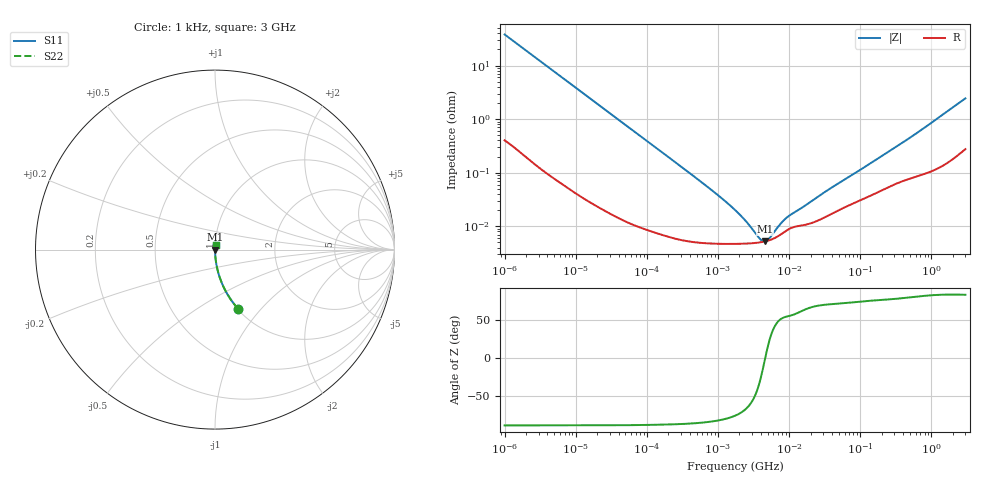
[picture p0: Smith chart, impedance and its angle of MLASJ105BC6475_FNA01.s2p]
! MLASJ105BC6475_FNA01  S-PARAMETER MODEL  ( Standard Model )
! Model Generated by TAIYO YUDEN Corporation (http://www.ty-top.com)
! Version 1.0
! TAIYO YUDEN Control No. 220601
! Copyright(c) 2013 TAIYO YUDEN CO.,LTD. All Rights Reserved.
! Product Description (link to TY-COMPAS)
! https://ds.yuden.co.jp/TYCOMPAS/or/detail?pn=MLASJ105BC6475MFNA01&u=M
! Products Name : Multilayer Ceramic Capacitors
! Characteristics :
!  Capacitance : 4.7 [uF] , Rated Voltage : 6.3 [V] , TCC : X6S
!  Case Size : 1.0 x 0.5 / 0.039 x 0.02 [mm/inch] , Thickness : 0.5 / 0.02 [mm/inch]
!  (Conditions: Temperature = 25 [degC] , DC Bias Voltage = 0 [V])
! External Node Assignments :
!  1  o---| |---o  2
! GND o---------o GND
! Frequency Range : 1kHz  -  3GHz  [ 401 STEP ]
# MHZ S RI R 50
! Freq[MHz].  S11 Real  S11 Imag  S21 Real  S21 Imag  S12 Real  S12 Imag  S22 Real  S22 Imag
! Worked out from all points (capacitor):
!   401 points, 1 kHz to 3 GHz, reference 50 ohm
!   read as one part in series: C = 4.18 uF near 1.077 kHz
!   lowest |Z| = 5.21 mohm at 4.566 MHz (marker M1)
!   series resonance near 4.61 MHz, so ESL is about 280 pH
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0.001  0.1285 -0.3294  0.8715 0.3294  0.8715 0.3294  0.1285 -0.3294
0.001685  0.0507 -0.2142  0.9493 0.2142  0.9493 0.2142  0.0507 -0.2142
0.00306  0.0166 -0.1228  0.9834 0.1228  0.9834 0.1228  0.0166 -0.1228
0.005768  0.00508 -0.0662  0.9949 0.0662  0.9949 0.0662  0.00508 -0.0662
0.01216  0.00135 -0.0317  0.9986 0.0317  0.9986 0.0317  0.00135 -0.0317
0.033275  0.000297 -0.0117  0.9997 0.0117  0.9997 0.0117  0.000297 -0.0117
0.147855  7.91e-05 -0.00265  0.9999 0.00265  0.9999 0.00265  7.91e-05 -0.00265
0.762639  4.81e-05 -0.000504  1 0.000504  1 0.000504  4.81e-05 -0.000504
1.238299  4.7e-05 -0.000297  1 0.000297  1 0.000297  4.7e-05 -0.000297
1.732051  4.7e-05 -0.000197  1 0.000197  1 0.000197  4.7e-05 -0.000197
2.812335  4.8e-05 -8.88e-05  1 8.88e-05  1 8.88e-05  4.8e-05 -8.88e-05
3.03007  4.83e-05 -7.46e-05  1 7.46e-05  1 7.46e-05  4.83e-05 -7.46e-05
4.566395  5.21e-05 -1.63e-06  0.9999 1.63e-06  0.9999 1.63e-06  5.21e-05 -1.63e-06
6.881678  6.46e-05 7.03e-05  0.9999 -7.03e-05  0.9999 -7.03e-05  6.46e-05 7.03e-05
7.414467  6.87e-05 8.33e-05  0.9999 -8.33e-05  0.9999 -8.33e-05  6.87e-05 8.33e-05
9.991309  8.92e-05 0.00013  0.9999 -0.00013  0.9999 -0.00013  8.92e-05 0.00013
21.06097  0.000116 0.000277  0.9999 -0.000277  0.9999 -0.000277  0.000116 0.000277
38.244  0.000167 0.000485  0.9998 -0.000485  0.9998 -0.000485  0.000167 0.000485
256.0921  0.000554 0.00246  0.9994 -0.00246  0.9994 -0.00246  0.000554 0.00246
603.7133  0.000867 0.00527  0.9991 -0.00527  0.9991 -0.00527  0.000867 0.00527
2784.426  0.00304 0.0225  0.997 -0.0225  0.997 -0.0225  0.00304 0.0225
3000  0.00333 0.0241  0.9967 -0.0241  0.9967 -0.0241  0.00333 0.0241
